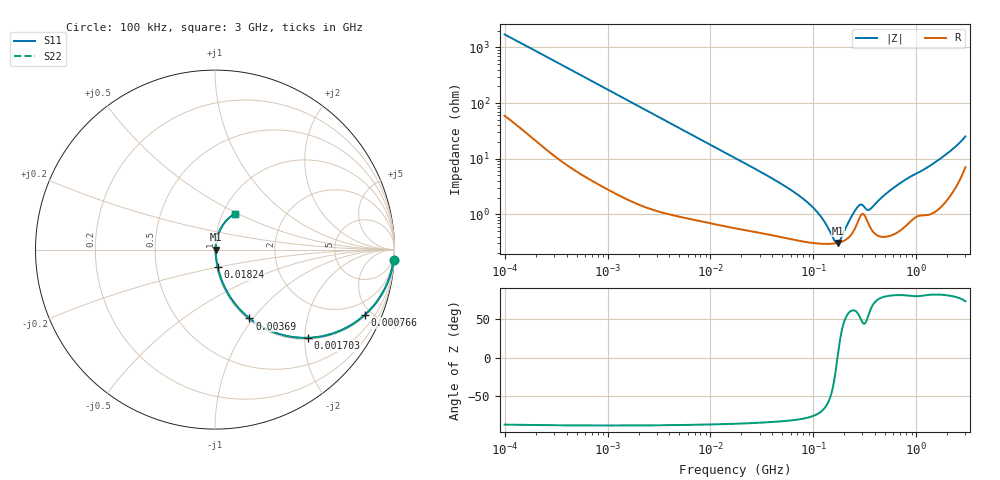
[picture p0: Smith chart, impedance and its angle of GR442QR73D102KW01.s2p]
!Murata Part Number: GR442QR73D102KW01
!These Parameters are Measured in Series Mode Connection
!Data Generated on Mar 13, 2026
!  o--ll--o
!Port1  Port2
!  o------o
!Operation Temp=25[degC], DC Bias Voltage=0[V]
!Freq. Start=100[kHz] Stop=3[GHz] 401[Steps]
# Hz S RI R 50
!Freq.(Hz) S11(Real) S11(Imag) S21(Real) S21(Imag) S12(Real) S12(Imag) S22(Real) S22(Imag)
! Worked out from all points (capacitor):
!   401 points, 100 kHz to 3 GHz, reference 50 ohm
!   read as one part in series: C = 926 pF near 105.3 kHz
!   lowest |Z| = 306 mohm at 171.7 MHz (marker M1)
!   series resonance near 171.6 MHz, so ESL is about 930 pH
!   S11 on the Smith chart (normalised r, x): 100 kHz: 2, -34; 766 kHz: 1.07, -4.57; 1.703 MHz: 1.03, -2.07; 3.69 MHz: 1.02, -0.96; 18.24 MHz: 1.01, -0.20; 3 GHz: 1.14, +0.48
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100000  0.9946 -0.0581  0.00541 0.0581  0.00541 0.0581  0.9946 -0.0581
252895  0.9763 -0.1417  0.0237 0.1417  0.0237 0.1417  0.9763 -0.1417
562235  0.9022 -0.2888  0.0978 0.2888  0.0978 0.2888  0.9022 -0.2888
766005  0.8354 -0.3629  0.1646 0.3629  0.1646 0.3629  0.8354 -0.3629
1702975  0.5164 -0.4915  0.4836 0.4915  0.4836 0.4915  0.5164 -0.4915
3161081  0.2425 -0.4187  0.7575 0.4187  0.7575 0.4187  0.2425 -0.4187
3689712  0.192 -0.3833  0.808 0.3833  0.808 0.3833  0.192 -0.3833
7027689  0.0666 -0.2342  0.9334 0.2342  0.9334 0.2342  0.0666 -0.2342
1.77727e7  0.0154 -0.0985  0.9846 0.0985  0.9846 0.0985  0.0154 -0.0985
1.82367e7  0.0148 -0.096  0.9852 0.096  0.9852 0.096  0.0148 -0.096
5.523785e7  0.00461 -0.0302  0.9954 0.0302  0.9954 0.0302  0.00461 -0.0302
9.738194e7  0.00324 -0.0133  0.9968 0.0133  0.9968 0.0133  0.00324 -0.0133
1.196798e8  0.00302 -0.00832  0.997 0.00832  0.997 0.00832  0.00302 -0.00832
1.589065e8  0.00299 -0.00179  0.997 0.00179  0.997 0.00179  0.00299 -0.00179
1.716802e8  0.00306 9.1e-06  0.9969 -9.1e-06  0.9969 -9.1e-06  0.00306 9.1e-06
1.854806e8  0.00318 0.00185  0.9968 -0.00185  0.9968 -0.00185  0.00318 0.00185
2.339019e8  0.00438 0.00786  0.9956 -0.00786  0.9956 -0.00786  0.00438 0.00786
2.730175e8  0.0077 0.0116  0.9923 -0.0116  0.9923 -0.0116  0.0077 0.0116
3.532796e8  0.00614 0.0106  0.9939 -0.0106  0.9939 -0.0106  0.00614 0.0106
5.475153e8  0.00472 0.0257  0.9953 -0.0257  0.9953 -0.0257  0.00472 0.0257
1.838476e9  0.0262 0.105  0.9738 -0.105  0.9738 -0.105  0.0262 0.105
3e9  0.1109 0.2007  0.8891 -0.2007  0.8891 -0.2007  0.1109 0.2007
